[IBIS ver]   3.2
[Comment char]  |_char
[File name]   35a302b_mi001_04.ibs
[File Rev]   1.3
[Date]   08-14-2003
[Notes]
|   Revision History:
|   1.0  08-14-03 Initial release.
|   1.1  02-20-04 Fixed comments for package to 456
|   1.2  04-04-05 Fixed Rref value to 1K from 1E20K
|   1.3  08-31-09 Updated with IDT formatting
[Disclaimer] This model is subject to change.
   Integrated Device Technology, Inc. ("IDT") hereby grants the
   user of this IBIS model a non-exclusive, nontransferable
   license to use this IBIS model under the following terms. The
   user is granted this license only to use the IBIS model and is
   not granted rights to sell, copy (except as needed to run the
   IBIS model), rent, lease or sub-license the IBIS model in
   whole or in part, or in modified form to anyone. The User may
   modify the IBIS model to suit its specific applications, but
   rights to derivative works and such modifications shall belong
   to IDT. This IBIS model is provided on an AS IS" basis and IDT
   makes absolutely no warranty with respect to the information
   contained herein. IDT DISCLAIMS AND CUSTOMER WAIVES ALL
   WARRANTIES, EXPRESS AND IMPLIED, INCLUDING WARRANTIES OF
   MERCHANTABILITY AND FITNESS FOR A PARTICULAR PURPOSE. THE
   ENTIRE RISK AS TO QUALITY AND PERFORMANCE IS WITH THE USER
   ACCORDINGLY, IN NO EVENT SHALL IDT BE LIABLE FOR ANY DIRECT OR
   INDIRECT DAMAGES, WHETHER IN CONTRACT OR TORT, INCLUDING ANY
   LOST PROFITS OR OTHER INCIDENTAL, CONSEQUENTIAL, EXEMPLARY, OR
   PUNITIVE DAMAGES ARISING OUT OF THE USE OR APPLICATION OF THE
   IBIS model. Further, IDT reserves the right to make changes
   without notice to any product herein to improve reliability,
   function, or design. IDT does not convey any license under
   patent rights or any other intellectual property rights,
   including those of third parties. IDT is not obligated to
   provide maintenance or support for the licensed IBIS model.
[Copyright]   Copyright 2009, Integrated Device Technology, Inc. all
   rights reserved.
|   This is the IBIS model for the Tsi148 chip.
|   456 PBGA.
|   Component Tsi148
[Component]   Tsi148
[Manufacturer]   Integrated Device Technology, Inc.
[Package]
|  variable   typ   min   max
R_pkg   0.30ohm   0.252ohm   0.440ohm
L_pkg   8.00nH   5.722nH   11.199nH
C_pkg   0.50pF   0.346pF   0.774pF
|Package parameters for Lead including bondwires
[Pin]   signal_name   model_name   R_pin   L_pin   C_pin
AF5   CBE0_L   bpcix3cppu_a   0.379   9.428nH   0.374pF
AD6   CBE1_L   bpcix3cppu_a   0.324   7.577nH   0.434pF
AE6   CBE2_L   bpcix3cppu_a   0.355   8.537nH   0.413pF
AF4   CBE3_L   bpcix3cppu_a   0.382   9.849nH   0.357pF
AA3   CBE4_L   bpcix3cppu_a   0.322   7.624nH   0.414pF
AB1   CBE5_L   bpcix3cppu_a   0.373   9.578nH   0.386pF
Y2   CBE6_L   bpcix3cppu_a   0.318   7.924nH   0.451pF
Y3   CBE7_L   bpcix3cppu_a   0.292   7.276nH   0.451pF
AE3   FRAME_L   bpcix3cppu_a   0.356   9.677nH   0.482pF
AD5   IRDY_L   bpcix3cppu_a   0.309   7.581nH   0.488pF
AF3   TRDY_L   bpcix3cppu_a   0.392   9.884nH   0.406pF
AE4   STOP_L   bpcix3cppu_a   0.373   9.130nH   0.402pF
AF2   DEVSEL_L   bpcix3cppu_a   0.364   10.624nH  0.544pF
AE5   IDSEL   bpcix3cppu_a   0.350   8.238nH   0.409pF
AC1   REQ64_L   bpcix3cppu_a   0.367   9.570nH   0.385pF
AA2   ACK64_L   bpcix3cppu_a   0.346   8.353nH   0.419pF
AE7   PAR   bpcix3cppu_a   0.350   8.344nH   0.458pF
W2   PAR64   bpcix3cppu_a   0.327   8.285nH   0.464pF
AC2   SERR_L   bpcix3cppu_a   0.355   9.027nH   0.452pF
AB2   PERR_L   bpcix3cppu_a   0.334   8.218nH   0.417pF
AD2   REQ_L   bpcix3cppu_a   0.347   8.767nH   0.774pF
AB3   GNT_L   bpcix3cppu_a   0.293   7.165nH   0.557pF
AD1   M66EN   bpcix3cppu_a   0.377   9.657nH   0.463pF
F3   INTA_L   bt3335pu_a   0.322   7.815nH   0.449pF
E1   INTB_L   bt3335pu_a   0.375   9.556nH   0.385pF
G2   INTC_L   bt3335pu_a   0.347   8.279nH   0.414pF
G3   INTD_L   bt3335pu_a   0.317   7.565nH   0.417pF
Y24   BDFAIL_L   bt3365pu_a   0.353   8.112nH   0.470pF
W23   LRSTI_L   bt3365pu_a   0.318   7.006nH   0.522pF
W25   LRSTO_L   bt3365pu_a   0.369   8.741nH   0.499pF
Y26   LSRSTI_L   bt3365pu_a   0.383   9.448nH   0.446pF
W24   PURSTI_L   bt3365pu_a   0.332   7.580nH   0.481pF
D7   PCLK   bpcix3cppu_a   0.321   7.139nH   0.443pF
D2   TCK   bt3365pd_a   0.378   9.409nH   0.452pF
E2   TMS   bt3365pd_a   0.352   8.595nH   0.449pF
D1   TRST_L   bt3365pd_a   0.388   10.239nH  0.406pF
C1   TDI   bt3365pd_a   0.399   10.385nH  0.456pF
F2   TDO   bt3365pd_a   0.355   8.835nH   0.429pF
C5   PLL_OUTA   bc1865_a   0.326   8.120nH   0.405pF
A9   PLL_GNDA   GND   0.360   9.091nH   0.440pF
AD19   AD0   bpcix3cppu_a   0.289   7.558nH   0.489pF
AE18   AD1   bpcix3cppu_a   0.314   8.336nH   0.450pF
AF19   AD2   bpcix3cppu_a   0.338   9.330nH   0.410pF
AD18   AD3   bpcix3cppu_a   0.288   7.537nH   0.464pF
AE17   AD4   bpcix3cppu_a   0.305   8.040nH   0.452pF
AF18   AD5   bpcix3cppu_a   0.326   8.917nH   0.450pF
AD17   AD6   bpcix3cppu_a   0.282   7.257nH   0.478pF
AE16   AD7   bpcix3cppu_a   0.296   7.510nH   0.422pF
AD16   AD8   bpcix3cppu_a   0.284   6.997nH   0.403pF
AE15   AD9   bpcix3cppu_a   0.288   7.358nH   0.404pF
AD15   AD10   bpcix3cppu_a   0.277   6.781nH   0.405pF
AE14   AD11   bpcix3cppu_a   0.300   7.516nH   0.382pF
AF15   AD12   bpcix3cppu_a   0.321   8.340nH   0.360pF
AF14   AD13   bpcix3cppu_a   0.300   7.754nH   0.372pF
AD13   AD14   bpcix3cppu_a   0.257   6.224nH   0.426pF
AD14   AD15   bpcix3cppu_a   0.275   6.779nH   0.428pF
AF13   AD16   bpcix3cppu_a   0.306   8.030nH   0.364pF
AE13   AD17   bpcix3cppu_a   0.296   7.577nH   0.422pF
AD12   AD18   bpcix3cppu_a   0.278   6.782nH   0.391pF
AE12   AD19   bpcix3cppu_a   0.299   7.528nH   0.397pF
AD11   AD20   bpcix3cppu_a   0.282   6.894nH   0.431pF
AF10   AD21   bpcix3cppu_a   0.305   8.113nH   0.457pF
AE11   AD22   bpcix3cppu_a   0.286   7.172nH   0.433pF
AD10   AD23   bpcix3cppu_a   0.271   6.530nH   0.421pF
AF9   AD24   bpcix3cppu_a   0.319   8.425nH   0.437pF
AD9   AD25   bpcix3cppu_a   0.297   7.164nH   0.473pF
AF8   AD26   bpcix3cppu_a   0.328   8.629nH   0.494pF
AE9   AD27   bpcix3cppu_a   0.322   8.208nH   0.549pF
AD8   AD28   bpcix3cppu_a   0.293   7.023nH   0.505pF
AF7   AD29   bpcix3cppu_a   0.355   9.211nH   0.431pF
AE8   AD30   bpcix3cppu_a   0.334   8.322nH   0.486pF
AD7   AD31   bpcix3cppu_a   0.319   7.610nH   0.457pF
Y1   AD32   bpcix3cppu_a   0.350   9.430nH   0.432pF
W3   AD33   bpcix3cppu_a   0.290   7.613nH   0.517pF
V2   AD34   bpcix3cppu_a   0.319   8.364nH   0.529pF
W1   AD35   bpcix3cppu_a   0.342   9.342nH   0.458pF
V3   AD36   bpcix3cppu_a   0.291   7.503nH   0.529pF
U2   AD37   bpcix3cppu_a   0.309   8.032nH   0.492pF
V1   AD38   bpcix3cppu_a   0.327   8.944nH   0.472pF
U3   AD39   bpcix3cppu_a   0.282   7.249nH   0.473pF
T2   AD40   bpcix3cppu_a   0.296   7.512nH   0.412pF
T3   AD41   bpcix3cppu_a   0.282   6.999nH   0.390pF
R2   AD42   bpcix3cppu_a   0.287   7.353nH   0.389pF
R3   AD43   bpcix3cppu_a   0.275   6.780nH   0.399pF
P2   AD44   bpcix3cppu_a   0.298   7.518nH   0.375pF
R1   AD45   bpcix3cppu_a   0.320   8.360nH   0.347pF
P1   AD46   bpcix3cppu_a   0.300   7.771nH   0.363pF
N3   AD47   bpcix3cppu_a   0.257   6.174nH   0.426pF
P3   AD48   bpcix3cppu_a   0.275   6.700nH   0.424pF
N1   AD49   bpcix3cppu_a   0.306   7.922nH   0.373pF
N2   AD50   bpcix3cppu_a   0.297   7.539nH   0.433pF
M3   AD51   bpcix3cppu_a   0.278   6.780nH   0.406pF
M2   AD52   bpcix3cppu_a   0.300   7.550nH   0.414pF
L3   AD53   bpcix3cppu_a   0.283   6.902nH   0.433pF
K1   AD54   bpcix3cppu_a   0.306   8.164nH   0.463pF
L2   AD55   bpcix3cppu_a   0.286   7.230nH   0.440pF
K3   AD56   bpcix3cppu_a   0.271   6.566nH   0.414pF
J1   AD57   bpcix3cppu_a   0.320   8.497nH   0.424pF
J3   AD58   bpcix3cppu_a   0.298   7.210nH   0.481pF
H1   AD59   bpcix3cppu_a   0.329   8.750nH   0.495pF
J2   AD60   bpcix3cppu_a   0.322   8.311nH   0.558pF
H3   AD61   bpcix3cppu_a   0.293   7.110nH   0.486pF
G1   AD62   bpcix3cppu_a   0.354   9.347nH   0.402pF
H2   AD63   bpcix3cppu_a   0.335   8.396nH   0.449pF
K24   VA1   bt3335pu_a   0.314   7.468nH   0.463pF
L25   VA2   bt3335pu_a   0.335   8.099nH   0.423pF
K26   VA3   bt3335pu_a   0.345   8.699nH   0.382pF
L23   VA4   bt3335pu_a   0.290   6.634nH   0.441pF
L24   VA5   bt3335pu_a   0.313   7.329nH   0.424pF
M25   VA6   bt3335pu_a   0.322   7.711nH   0.428pF
N23   VA7   bt3335pu_a   0.294   6.701nH   0.448pF
M24   VA8   bt3335pu_a   0.316   7.287nH   0.431pF
M23   VA9   bt3335pu_a   0.253   5.722nH   0.464pF
N25   VA10   bt3335pu_a   0.328   7.822nH   0.428pF
M26   VA11   bt3335pu_a   0.349   8.600nH   0.391pF
N26   VA12   bt3335pu_a   0.316   7.886nH   0.371pF
P24   VA13   bt3335pu_a   0.285   6.621nH   0.383pF
N24   VA14   bt3335pu_a   0.310   7.182nH   0.389pF
P26   VA15   bt3335pu_a   0.339   8.405nH   0.346pF
R26   VA16   bt3335pu_a   0.352   8.674nH   0.357pF
P25   VA17   bt3335pu_a   0.331   7.857nH   0.372pF
R24   VA18   bt3335pu_a   0.298   6.940nH   0.399pF
R23   VA19   bt3335pu_a   0.286   6.433nH   0.383pF
P23   VA20   bt3335pu_a   0.263   5.818nH   0.429pF
R25   VA21   bt3335pu_a   0.314   7.703nH   0.448pF
T24   VA22   bt3335pu_a   0.290   6.695nH   0.418pF
T23   VA23   bt3335pu_a   0.298   6.830nH   0.456pF
U26   VA24   bt3335pu_a   0.356   8.847nH   0.411pF
T25   VA25   bt3335pu_a   0.351   8.311nH   0.445pF
U24   VA26   bt3335pu_a   0.325   7.522nH   0.474pF
V26   VA27   bt3335pu_a   0.360   9.161nH   0.445pF
U23   VA28   bt3335pu_a   0.307   6.868nH   0.460pF
U25   VA29   bt3335pu_a   0.360   8.593nH   0.445pF
V24   VA30   bt3335pu_a   0.322   7.490nH   0.458pF
W26   VA31   bt3335pu_a   0.374   9.574nH   0.442pF
D6   VD0   bt3335pu_a   0.342   7.761nH   0.496pF
A4   VD1   bt3335pu_a   0.409   10.287nH  0.392pF
B6   VD2   bt3335pu_a   0.390   9.121nH   0.457pF
B7   VD3   bt3335pu_a   0.381   8.919nH   0.495pF
C7   VD4   bt3335pu_a   0.343   7.952nH   0.494pF
D8   VD5   bt3335pu_a   0.328   7.239nH   0.500pF
D9   VD6   bt3335pu_a   0.313   6.980nH   0.470pF
B9   VD7   bt3335pu_a   0.354   8.500nH   0.452pF
A8   VD8   bt3335pu_a   0.381   9.762nH   0.431pF
C9   VD9   bt3335pu_a   0.323   7.731nH   0.460pF
B10   VD10   bt3335pu_a   0.333   8.122nH   0.442pF
B11   VD11   bt3335pu_a   0.336   8.145nH   0.444pF
A10   VD12   bt3335pu_a   0.346   8.747nH   0.405pF
D11   VD13   bt3335pu_a   0.290   6.647nH   0.434pF
C11   VD14   bt3335pu_a   0.313   7.369nH   0.416pF
B12   VD15   bt3335pu_a   0.322   7.787nH   0.421pF
D13   VD16   bt3335pu_a   0.293   6.726nH   0.428pF
C12   VD17   bt3335pu_a   0.315   7.309nH   0.423pF
D12   VD18   bt3335pu_a   0.252   5.737nH   0.445pF
B13   VD19   bt3335pu_a   0.327   7.853nH   0.406pF
A12   VD20   bt3335pu_a   0.349   8.662nH   0.368pF
A13   VD21   bt3335pu_a   0.317   7.903nH   0.376pF
C14   VD22   bt3335pu_a   0.285   6.607nH   0.391pF
C13   VD23   bt3335pu_a   0.309   7.158nH   0.405pF
A14   VD24   bt3335pu_a   0.338   8.316nH   0.369pF
A15   VD25   bt3335pu_a   0.352   8.556nH   0.368pF
B14   VD26   bt3335pu_a   0.331   7.810nH   0.393pF
C15   VD27   bt3335pu_a   0.298   6.922nH   0.413pF
D15   VD28   bt3335pu_a   0.286   6.396nH   0.386pF
D14   VD29   bt3335pu_a   0.263   5.764nH   0.432pF
B15   VD30   bt3335pu_a   0.313   7.666nH   0.447pF
C16   VD31   bt3335pu_a   0.290   6.647nH   0.418pF
H24   AM0   bt3335pu_a   0.338   7.869nH   0.492pF
J23   AM1   bt3335pu_a   0.313   6.960nH   0.443pF
J25   AM2   bt3335pu_a   0.354   8.491nH   0.440pF
H26   AM3   bt3335pu_a   0.380   9.768nH   0.437pF
J24   AM4   bt3335pu_a   0.323   7.735nH   0.459pF
K25   AM5   bt3335pu_a   0.333   8.132nH   0.422pF
G26   IACK_L   bt3335pu_a   0.386   9.569nH   0.464pF
J26   LWORD_L   bt3335pu_a   0.359   9.115nH   0.417pF
K23   WRITE_L   bt3335pu_a   0.297   6.732nH   0.443pF
G23   ASI_L   bt3365pu_a   0.332   7.239nH   0.467pF
F24   ASO_L   bt3335pu_a   0.372   8.521nH   0.473pF
E25   DS0I_L   bt3365pu_a   0.373   8.962nH   0.469pF
D25   DS0O_L   bt3335pu_a   0.397   9.652nH   0.466pF
D26   DS1I_L   bt3365pu_a   0.440   10.418nH  0.440pF
F23   DS1O_L   bt3335pu_a   0.348   7.775nH   0.498pF
E23   DTACKI_L   ip33d2t_a   0.324   7.754nH   0.606pF
D24   DTACKO_L   bt3335pu_a   0.378   9.231nH   0.473pF
H25   RETRYI_L   bt3365pu_a   0.382   8.916nH   0.458pF
H23   RETRYO_L   bt3335pu_a   0.331   7.276nH   0.472pF
C22   BERRI_L   bt3365pu_a   0.351   8.326nH   0.462pF
A24   BERRO_L   bt3335pu_a   0.436   11.103nH  0.423pF
D20   BR0I_L   bp3365_a   0.337   7.739nH   0.478pF
C21   BR1I_L   bp3365_a   0.365   8.557nH   0.475pF
A23   BR2I_L   bp3365_a   0.423   10.548nH  0.458pF
B22   BR3I_L   bp3365_a   0.373   8.906nH   0.491pF
B20   BR0O   bt3335pd_a   0.382   9.099nH   0.473pF
A22   BR1O   bt3335pd_a   0.400   10.026nH  0.434pF
B21   BR2O   bt3335pd_a   0.382   9.102nH   0.493pF
D21   BR3O   bt3335pd_a   0.355   7.981nH   0.500pF
B17   BG0IN_L   bp3365_a   0.359   8.574nH   0.430pF
B18   BG1IN_L   bp3365_a   0.355   8.605nH   0.484pF
A20   BG2IN_L   bp3365_a   0.383   9.575nH   0.427pF
C20   BG3IN_L   bp3365_a   0.354   8.244nH   0.466pF
D17   BG0INOUT_L   bp3335_a   0.306   6.889nH   0.439pF
A19   BG1INOUT_L   bp3335_a   0.374   9.559nH   0.463pF
C19   BG2INOUT_L   bp3335_a   0.330   7.630nH   0.462pF
D19   BG3INOUT_L   bp3335_a   0.318   7.097nH   0.501pF
A18   BG0OUT_L   bp3335_a   0.358   9.192nH   0.438pF
C18   BG1OUT_L   bp3335_a   0.322   7.456nH   0.473pF
D18   BG2OUT_L   bp3335_a   0.315   6.987nH   0.487pF
B19   BG3OUT_L   bp3335_a   0.368   8.853nH   0.473pF
A17   BBSYI_L   bt3365pu_a   0.356   8.835nH   0.402pF
D16   BBSYO   bt3335pd_a   0.297   6.793nH   0.456pF
C17   BCLRI_L   bt3365pu_a   0.324   7.528nH   0.458pF
B16   BCLRO_L   bt3335pu_a   0.351   8.290nH   0.440pF
G25   IACKIN_L   bp3365_a   0.383   9.031nH   0.462pF
E26   IACKOUT_L   bp3335_a   0.422   10.285nH  0.409pF
AA25   IRQ1I_L   ip33d1t_a   0.383   8.853nH   0.462pF
AC25   IRQ2I_L   bp3365_a   0.403   9.686nH   0.486pF
AB24   IRQ3I_L   bp3365_a   0.349   8.102nH   0.499pF
AD25   IRQ4I_L   ip33rit_a   0.403   9.561nH   0.588pF
AD23   IRQ5I_L   bp3365_a   0.330   8.591nH   0.573pF
AE23   IRQ6I_L   bp3365_a   0.362   9.215nH   0.540pF
AE21   IRQ7I_L   bp3365_a   0.352   8.437nH   0.514pF
AC26   IRQ1O   bt3365pd_a   0.424   10.353nH  0.425pF
AA23   IRQ2O   bt3365pd_a   0.353   7.847nH   0.492pF
AD26   IRQ3O   bt3365pd_a   0.435   10.782nH  0.444pF
AC24   IRQ4O   bt3365pd_a   0.381   8.954nH   0.553pF
AD22   IRQ5O   bt3365pd_a   0.294   7.551nH   0.603pF
AF24   IRQ6O   bt3365pd_a   0.387   10.287nH  0.508pF
AF23   IRQ7O   bt3365pd_a   0.372   9.636nH   0.471pF
AB26   SRSTI_L   bp3365_a   0.399   9.737nH   0.407pF
Y25   SRSTO   bt3365pd_a   0.382   8.904nH   0.476pF
AA24   SFAILI_L   bp3365_a   0.364   8.357nH   0.433pF
Y23   SFAILO   bt3365pd_a   0.336   7.608nH   0.445pF
V23   ACFAILI_L   bp3365_a   0.315   6.953nH   0.477pF
B24   AMOUT   bt3335pd_a   0.407   10.157nH  0.468pF
D22   DBOUT   bt3335pd_a   0.321   7.764nH   0.570pF
C23   DBOE_L   bt3335pu_a   0.384   9.308nH   0.472pF
A25   ADBOUT   bt3335pd_a   0.414   10.590nH  0.424pF
F25   ASOE   bt3335pd_a   0.414   9.407nH   0.475pF
C26   DSOE   bt3335pd_a   0.430   11.059nH  0.414pF
B23   BERROE   bt3335pd_a   0.407   9.891nH   0.469pF
C25   DTACKOE   bt3335pd_a   0.393   9.670nH   0.486pF
G24   RETRYOE   bt3335pd_a   0.345   8.019nH   0.483pF
AF22   GA0_L   bt3365pu_a   0.376   9.582nH   0.479pF
AE20   GA1_L   bt3365pu_a   0.323   7.913nH   0.492pF
AD20   GA2_L   bt3365pu_a   0.298   7.250nH   0.522pF
AE19   GA3_L   bt3365pu_a   0.328   8.266nH   0.431pF
AF20   GA4_L   bt3365pu_a   0.349   9.408nH   0.403pF
AD21   GAP_L   bt3365pu_a   0.328   7.720nH   0.509pF
E3   SCONEN_L   bt3365pu_a   0.307   7.584nH   0.543pF
C2   SCONDIS_L   bt3365pu_a   0.365   9.567nH   0.575pF
B1   SCON   bt3365pd_a   0.371   10.647nH  0.647pF
E24   SYSCLK   bt3335pu_a   0.335   8.091nH   0.464pF
B3   PLL_TUNE9   bt3365pu_a   0.380   9.986nH   0.483pF
A7   PLL_VDDA   POWER   0.385   9.525nH   0.513pF
B4   PLL_TUNE6   bt3365pu_a   0.390   9.684nH   0.445pF
C4   PLL_TUNE8   bt3365pu_a   0.364   9.225nH   0.434pF
C6   PLL_TUNE5   bt3365pu_a   0.358   8.299nH   0.436pF
A3   PLL_TUNE7   bt3365pu_a   0.422   11.199nH  0.390pF
C8   PLL_TUNE2   bt3365pu_a   0.339   7.873nH   0.534pF
A5   PLL_TUNE4   bt3365pu_a   0.417   10.084nH  0.398pF
D10   PLL_TUNE1   bt3365pu_a   0.297   6.744nH   0.461pF
B8   PLL_TUNE3   bt3365pu_a   0.377   8.875nH   0.515pF
C10   PLL_TUNE0   bt3365pu_a   0.315   7.472nH   0.483pF
D5   PLL_RSTI_L   bt3365pu_a   0.337   7.701nH   0.607pF
B5   PLL_TEN   bt3365pd_a   0.374   9.001nH   0.444pF
AB25   PCIMC   ip33mct_a   0.368   8.686nH   0.496pF
AC3   PCIPUEN   bt3365pd_a   0.326   7.937nH   0.562pF
AE22   CE0_TEST   ic18tepdt_a   0.338   8.304nH   0.510pF
AD4   HWC_PFU   bt3365pd_a   0.330   8.224nH   0.452pF
E5   VDD   POWER
E10   VDD   POWER
E11   VDD   POWER
E12   VDD   POWER
E15   VDD   POWER
E16   VDD   POWER
E17   VDD   POWER
E22   VDD   POWER
K5   VDD   POWER
K22   VDD   POWER
L5   VDD   POWER
L22   VDD   POWER
M5   VDD   POWER
M22   VDD   POWER
R5   VDD   POWER
R22   VDD   POWER
T5   VDD   POWER
T22   VDD   POWER
U5   VDD   POWER
U22   VDD   POWER
AB5   VDD   POWER
AB10   VDD   POWER
AB11   VDD   POWER
AB12   VDD   POWER
AB15   VDD   POWER
AB16   VDD   POWER
AB17   VDD   POWER
AB22   VDD   POWER
M14   VDD   POWER
N12   VDD   POWER
P15   VDD   POWER
R13   VDD   POWER
E4   VDD2   POWER
E6   VDD2   POWER
E7   VDD2   POWER
E8   VDD2   POWER
E13   VDD2   POWER
E19   VDD2   POWER
E20   VDD2   POWER
E21   VDD2   POWER
F4   VDD2   POWER
F5   VDD2   POWER
F22   VDD2   POWER
G4   VDD2   POWER
G5   VDD2   POWER
G22   VDD2   POWER
H4   VDD2   POWER
H5   VDD2   POWER
H22   VDD2   POWER
J4   VDD2   POWER
K4   VDD2   POWER
L4   VDD2   POWER
M4   VDD2   POWER
N4   VDD2   POWER
N22   VDD2   POWER
P4   VDD2   POWER
P5   VDD2   POWER
R4   VDD2   POWER
T4   VDD2   POWER
U4   VDD2   POWER
V4   VDD2   POWER
W4   VDD2   POWER
W5   VDD2   POWER
W22   VDD2   POWER
Y4   VDD2   POWER
Y5   VDD2   POWER
Y22   VDD2   POWER
AA4   VDD2   POWER
AA5   VDD2   POWER
AA22   VDD2   POWER
AB14   VDD2   POWER
AB19   VDD2   POWER
AB20   VDD2   POWER
AB21   VDD2   POWER
AB4   VDD2   POWER
AB6   VDD2   POWER
AB7   VDD2   POWER
AB8   VDD2   POWER
AC5   VDD2   POWER
AC6   VDD2   POWER
AC7   VDD2   POWER
AC8   VDD2   POWER
AC9   VDD2   POWER
AC10   VDD2   POWER
AC11   VDD2   POWER
AC12   VDD2   POWER
AC13   VDD2   POWER
AC14   VDD2   POWER
AC15   VDD2   POWER
AC16   VDD2   POWER
AC17   VDD2   POWER
AC18   VDD2   POWER
AC19   VDD2   POWER
AC20   VDD2   POWER
AC21   VDD2   POWER
AC22   VDD2   POWER
L12   VDD2   POWER
L15   VDD2   POWER
M11   VDD2   POWER
M16   VDD2   POWER
R11   VDD2   POWER
R16   VDD2   POWER
T12   VDD2   POWER
T15   VDD2   POWER
A1   VSS   GND
A2   VSS   GND
A6   VSS   GND
A11   VSS   GND
A16   VSS   GND
A21   VSS   GND
A26   VSS   GND
B2   VSS   GND
B25   VSS   GND
B26   VSS   GND
C3   VSS   GND
C24   VSS   GND
D4   VSS   GND
D23   VSS   GND
E9   VSS   GND
E14   VSS   GND
E18   VSS   GND
F1   VSS   GND
F26   VSS   GND
J5   VSS   GND
J22   VSS   GND
L1   VSS   GND
L26   VSS   GND
N5   VSS   GND
P22   VSS   GND
T1   VSS   GND
T26   VSS   GND
V5   VSS   GND
V22   VSS   GND
AA1   VSS   GND
AA26   VSS   GND
AB9   VSS   GND
AB13   VSS   GND
AB18   VSS   GND
AC4   VSS   GND
AC23   VSS   GND
AD3   VSS   GND
AD24   VSS   GND
AE1   VSS   GND
AE2   VSS   GND
AE25   VSS   GND
AF1   VSS   GND
AF6   VSS   GND
AF11   VSS   GND
AF16   VSS   GND
AF21   VSS   GND
AF25   VSS   GND
AF26   VSS   GND
L11   VSS   GND
L13   VSS   GND
L14   VSS   GND
L16   VSS   GND
M12   VSS   GND
M13   VSS   GND
M15   VSS   GND
N11   VSS   GND
N13   VSS   GND
N14   VSS   GND
N15   VSS   GND
N16   VSS   GND
P11   VSS   GND
P12   VSS   GND
P13   VSS   GND
P14   VSS   GND
P16   VSS   GND
R12   VSS   GND
R14   VSS   GND
R15   VSS   GND
T11   VSS   GND
T13   VSS   GND
T14   VSS   GND
T16   VSS   GND
[Model Selector]   bpcix3cppu_a
bpcix3cppu_a_mpa   Multiple Point Application
bpcix3cppu_a_ppa   Point to Point Application
[Submodel]  Up.ip33rit_a
Submodel_type   Dynamic_clamp
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[Submodel]  Dn.ip33rit_a
Submodel_type   Dynamic_clamp
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[Submodel]  Up.ip33d1t_a
Submodel_type   Dynamic_clamp
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[Submodel]  Dn.ip33d1t_a
Submodel_type   Dynamic_clamp
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[Submodel]  Up.ip33d2t_a
Submodel_type   Dynamic_clamp
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[Submodel]  Dn.ip33d2t_a
Submodel_type   Dynamic_clamp
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[Submodel]  Up.bp3365_a
Submodel_type   Dynamic_clamp
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[Submodel]  Up.bp3335_a
Submodel_type   Dynamic_clamp
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[Submodel]  Up.ip33mct_a
Submodel_type   Dynamic_clamp
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[Submodel]  Dn.ip33mct_a
Submodel_type   Dynamic_clamp
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| Models and submodels in the file (42): bpcix3cppu_a_mpa (I/O), Up.bpcix3cppu_a.mpa (Dynamic_clamp), Dn.bpcix3cppu_a.mpa (Dynamic_clamp), bpcix3cppu_a_ppa (I/O), Up.bpcix3cppu_a.ppa (Dynamic_clamp), Dn.bpcix3cppu_a.ppa (Dynamic_clamp), bt3335pu_a (I/O), Up.bt3335pu_a (Dynamic_clamp), Dn.bt3335pu_a (Dynamic_clamp), bt3365pu_a (I/O), Up.bt3365pu_a (Dynamic_clamp), Dn.bt3365pu_a (Dynamic_clamp), bt3365pd_a (I/O), Up.bt3365pd_a (Dynamic_clamp), Dn.bt3365pd_a (Dynamic_clamp), bc1865_a (I/O), Up.bc1865_a (Dynamic_clamp), Dn.bc1865_a (Dynamic_clamp), ip33rit_a (Input), Up.ip33rit_a (Dynamic_clamp), Dn.ip33rit_a (Dynamic_clamp), ip33d1t_a (Input), Up.ip33d1t_a (Dynamic_clamp), Dn.ip33d1t_a (Dynamic_clamp), ip33d2t_a (Input), Up.ip33d2t_a (Dynamic_clamp), Dn.ip33d2t_a (Dynamic_clamp), bp3365_a (I/O), Up.bp3365_a (Dynamic_clamp), Dn.bp3365_a (Dynamic_clamp), bp3335_a (I/O), Up.bp3335_a (Dynamic_clamp), Dn.bp3335_a (Dynamic_clamp), ic18tepdt_a (Input), Up.ic18tepdt_a (Dynamic_clamp), Dn.ic18tepdt_a (Dynamic_clamp), ip33mct_a (Input), Up.ip33mct_a (Dynamic_clamp), Dn.ip33mct_a (Dynamic_clamp), bt3335pd_a (I/O), Up.bt3335pd_a (Dynamic_clamp), Dn.bt3335pd_a (Dynamic_clamp)
